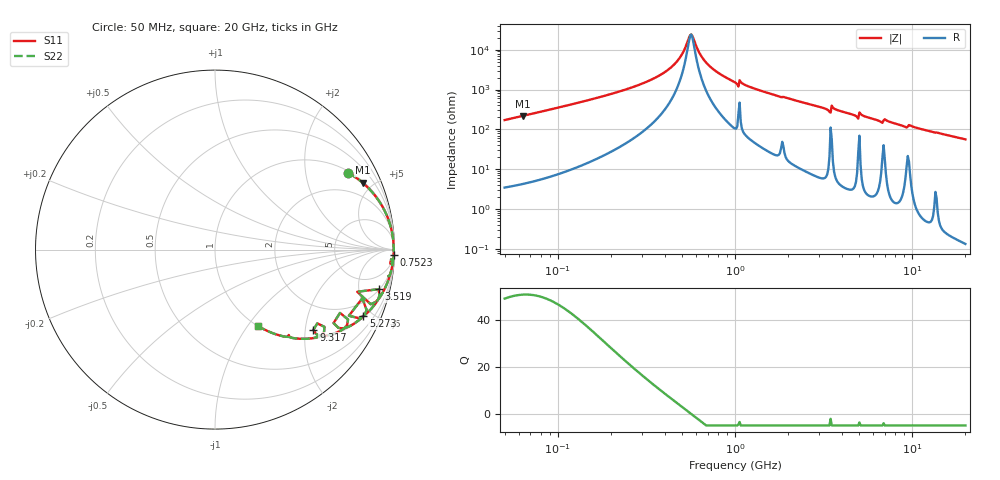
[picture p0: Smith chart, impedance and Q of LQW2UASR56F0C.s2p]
!Murata Part Number: LQW2UASR56F0C
!These Parameters are Measured in Series Mode Connection
!  o--[Z]--o
!Port1  Port2
!  o-------o
!Freq. Start=50[MHz] Stop=20[GHz], 401[Steps]
# Hz S RI R 50
!Freq.(Hz) S11(Real) S11(Imag) S21(Real) S21(Imag) S12(Real) S12(Imag) S22(Real) S22(Imag)
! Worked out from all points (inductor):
!   401 points, 50 MHz to 20 GHz, reference 50 ohm
!   read as one part in series: L = 541 nH near 51.52 MHz
!   highest Q = 51.1 at 63.54 MHz (marker M1), where L = 548 nH
!   self-resonance near 557.6 MHz
!   S11 on the Smith chart (normalised r, x): 50 MHz: 1.07, +3.43; 752.3 MHz: 10, -64; 3.519 GHz: 2.11, -7.84; 5.273 GHz: 1.08, -4.43; 9.317 GHz: 1.24, -2.21; 20 GHz: 1.00, -1.13
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5e7  0.7419 0.4276  0.2581 -0.4276  0.2581 -0.4276  0.7419 0.4276
6.354076e7  0.8224 0.3725  0.1776 -0.3725  0.1776 -0.3725  0.8224 0.3725
1.364002e8  0.9558 0.1933  0.0442 -0.1933  0.0442 -0.1933  0.9558 0.1933
2.520729e8  0.987 0.092  0.013 -0.092  0.013 -0.092  0.987 0.092
3.721004e8  0.9938 0.0444  0.00619 -0.0444  0.00619 -0.0444  0.9938 0.0444
4.728708e8  0.9955 0.0185  0.0045 -0.0185  0.0045 -0.0185  0.9955 0.0185
5.096456e8  0.9957 0.0107  0.00426 -0.0107  0.00426 -0.0107  0.9957 0.0107
5.492803e8  0.9959 0.00291  0.00415 -0.00291  0.00415 -0.00291  0.9959 0.00291
5.659842e8  0.9959 -0.000199  0.00413 0.000199  0.00413 0.000199  0.9959 -0.000199
6.476653e8  0.9957 -0.0142  0.00433 0.0142  0.00433 0.0142  0.9957 -0.0142
7.523192e8  0.995 -0.0302  0.00504 0.0302  0.00504 0.0302  0.995 -0.0302
1e9  0.9911 -0.0652  0.00886 0.0652  0.00886 0.0652  0.9911 -0.0652
2.728004e9  0.941 -0.227  0.059 0.227  0.059 0.227  0.941 -0.227
3.364474e9  0.8928 -0.2932  0.1072 0.2932  0.1072 0.2932  0.8928 -0.2932
3.519108e9  0.9126 -0.2205  0.0874 0.2205  0.0874 0.2205  0.9126 -0.2205
4.81993e9  0.8188 -0.3743  0.1812 0.3743  0.1812 0.3743  0.8188 -0.3743
5.273168e9  0.8266 -0.37  0.1734 0.37  0.1734 0.37  0.8266 -0.37
6.701223e9  0.688 -0.4361  0.312 0.4361  0.312 0.4361  0.688 -0.4361
7.442007e9  0.705 -0.4487  0.295 0.4487  0.295 0.4487  0.705 -0.4487
9.316812e9  0.5485 -0.4468  0.4515 0.4468  0.4515 0.4468  0.5485 -0.4468
1.201863e10  0.4725 -0.4967  0.5275 0.4967  0.5275 0.4967  0.4725 -0.4967
2e10  0.2413 -0.4267  0.7587 0.4267  0.7587 0.4267  0.2413 -0.4267
